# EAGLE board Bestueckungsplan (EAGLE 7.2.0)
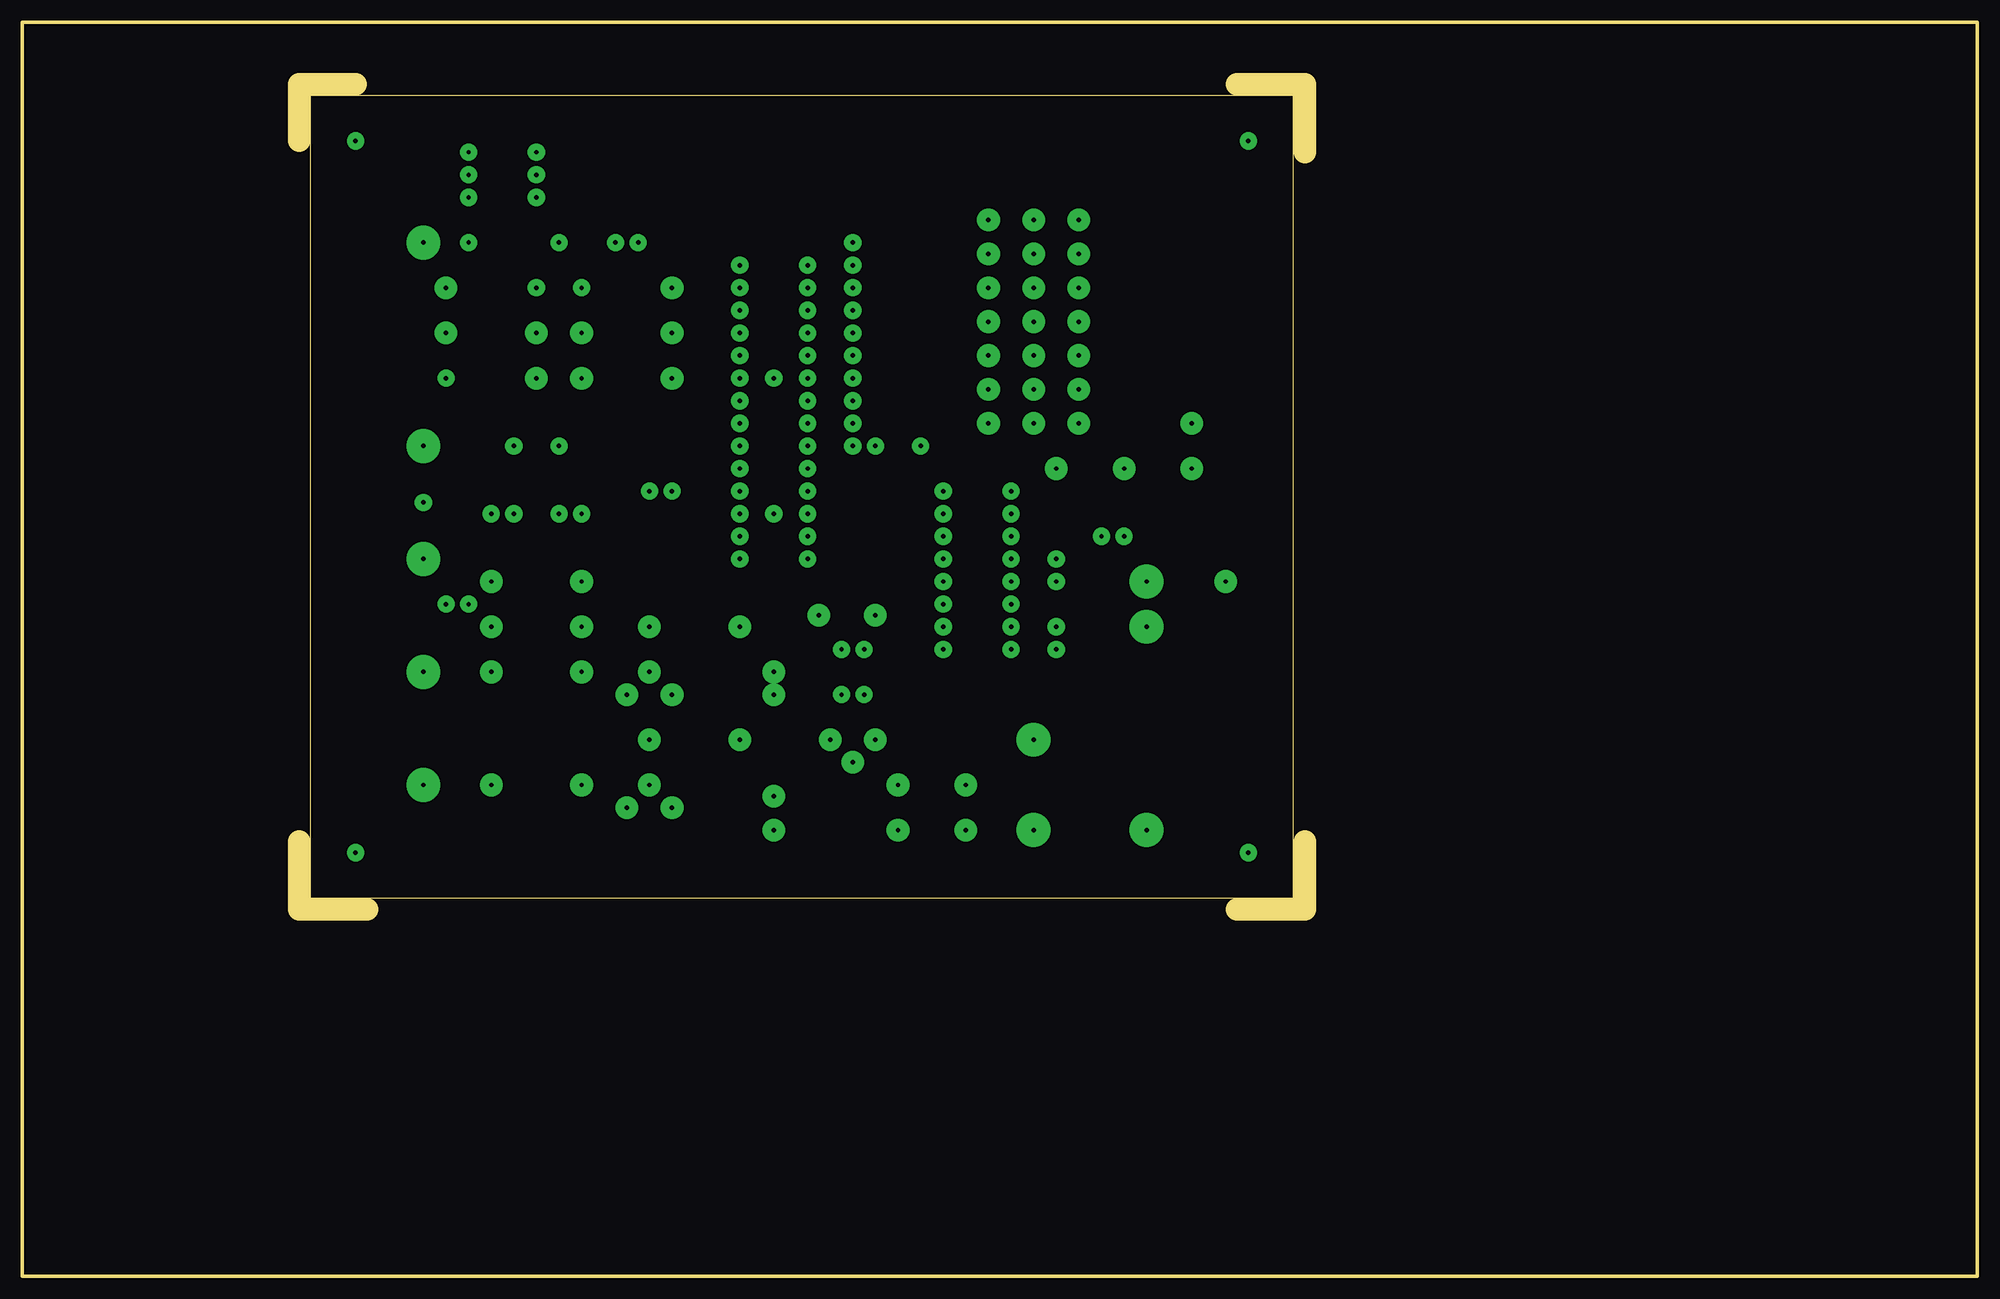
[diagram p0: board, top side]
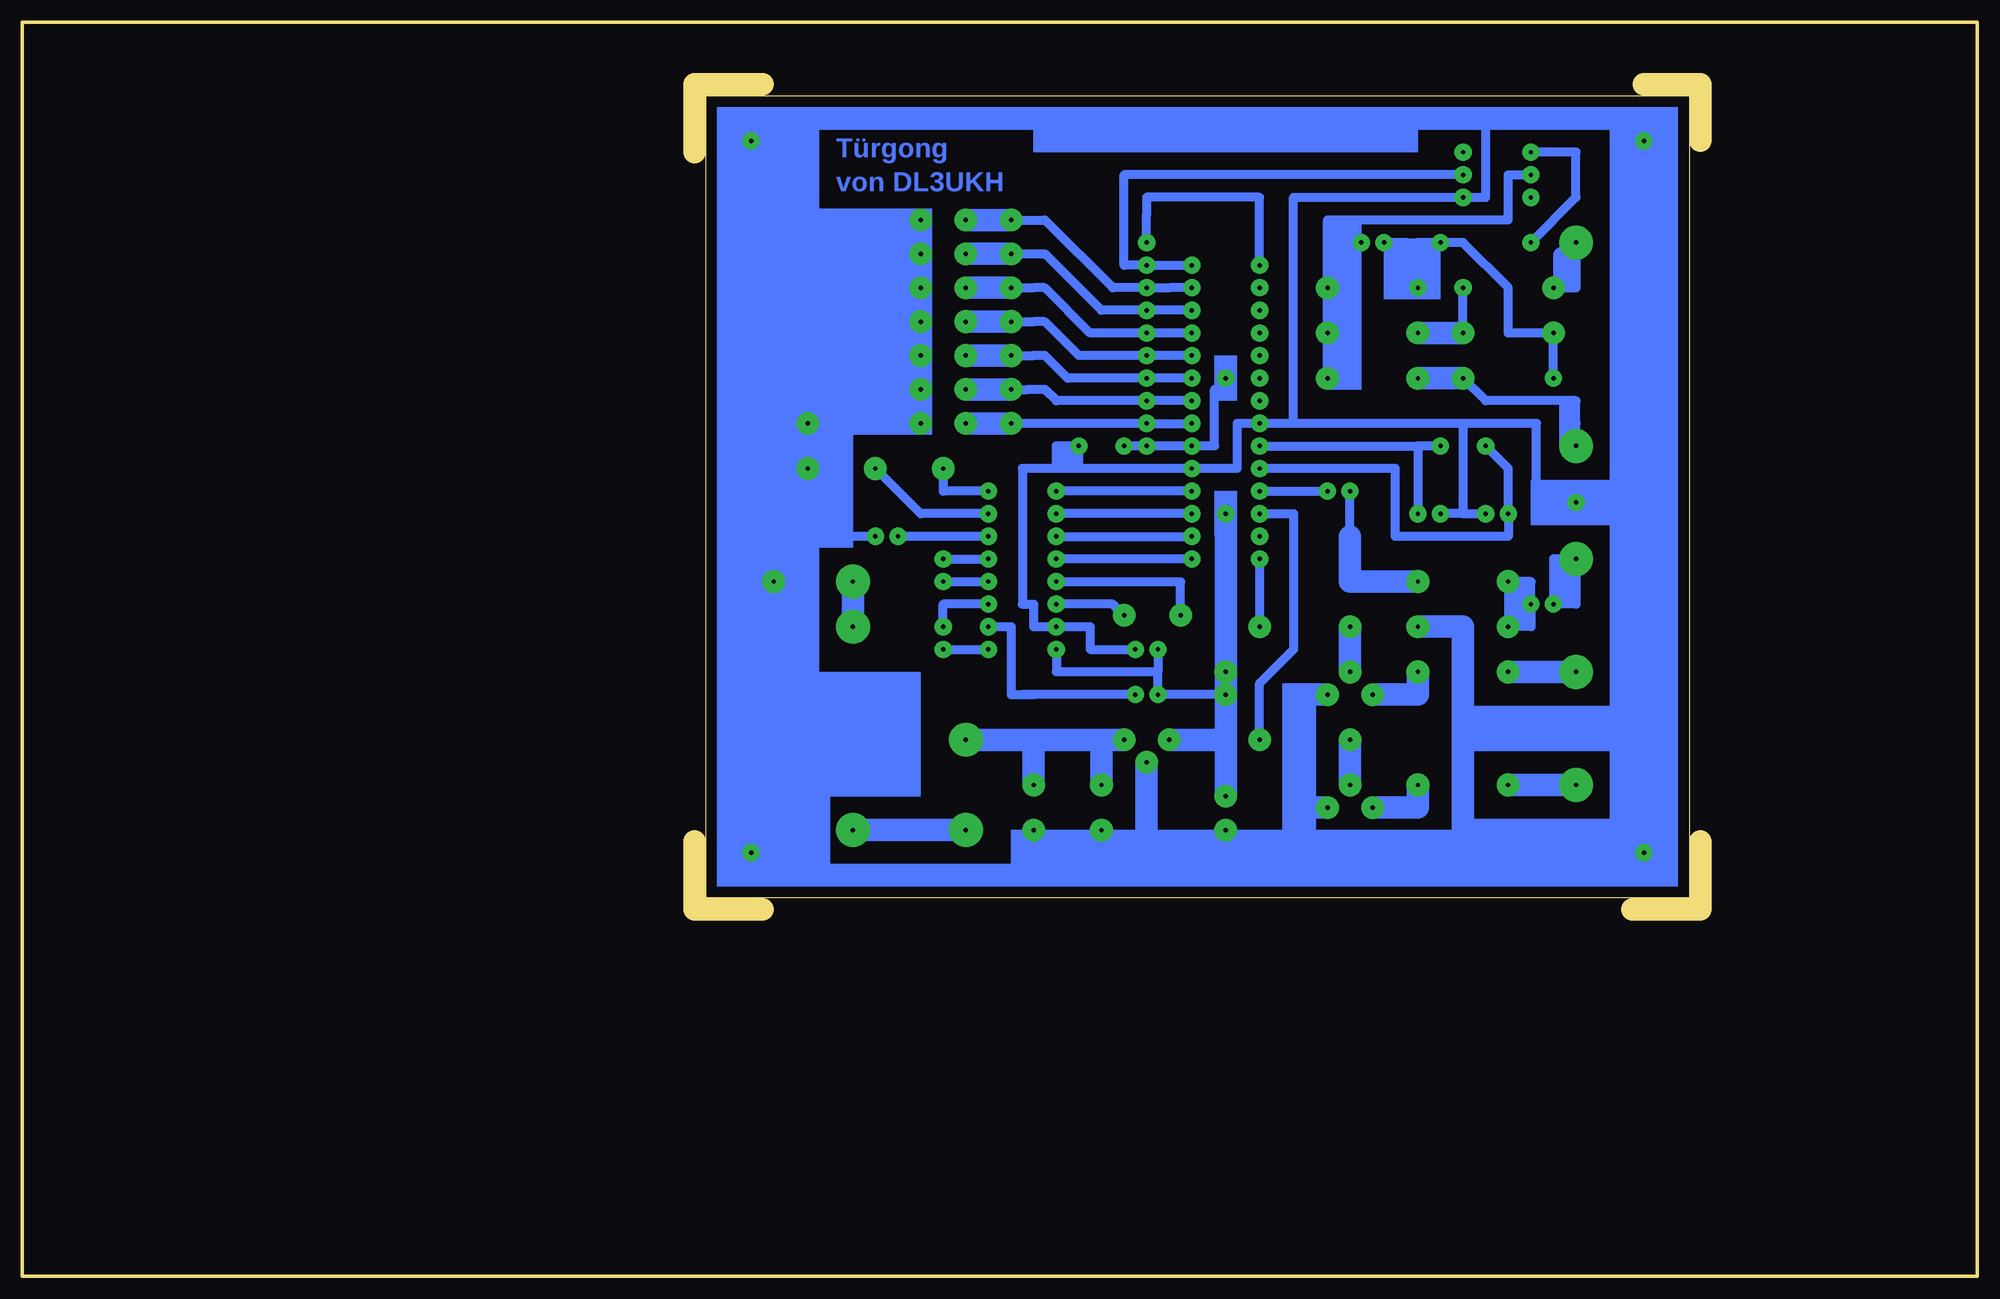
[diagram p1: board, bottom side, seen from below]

Size 219.71 x 140.97 mm. Coordinates in mm from the lower left corner, seen from the top.
Outline: 37.46,133.99 31.11,133.99 31.11,127.64
Outline: 136.53,133.99 144.15,133.99 144.15,126.36
Outline: 31.11,48.9 31.11,41.27 38.73,41.27
Outline: 136.53,41.27 144.15,41.27 144.15,48.9
Outline: 0,140.97 219.71,140.97 219.71,0 0,0 0,140.97
Outline: 32.38,42.55 142.88,42.55 142.88,132.72 32.38,132.72 32.38,42.55
Copper layers (1*16): Top 0.035mm / dielectric 1.5mm / Bottom 0.035mm
Design rules "default": minimum track width 10mil, minimum drill 24mil, track to track 8mil, track to pad 8mil, pad to pad 8mil, via to via 8mil, smd to smd 8mil, copper to edge 40mil, drill to drill 8mil, minimum pad ring 10mil, minimum via ring 8mil, stop-mask expansion 4mil, vias tented up to drill 0mil, thermal gap 10mil

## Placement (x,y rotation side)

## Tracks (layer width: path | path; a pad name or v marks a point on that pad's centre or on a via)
S$1  (via drill 0.5 pad 1.93, 0.5 pad 2.54)
  Bottom 1.016: v80.64,80.65 v80.64,73.03
S$2  (via drill 0.5 pad 1.93)
  other vias: 80.64,83.19
S$3  (via drill 0.5 pad 1.93, 0.5 pad 2.54)
  Bottom 1.016: v80.64,85.72 76.84,85.72 76.84,70.48 80.64,66.67 v80.64,60.33
S$4  (via drill 0.5 pad 2.54, 0.5 pad 3.81)
  Bottom 1.016: v45.08,116.2 45.08,111.12 v47.62,111.12
  Bottom 1.27: v45.08,116.2 46.99,114.94
S$5  (via drill 0.5 pad 1.93)
  Bottom 1.016: v80.64,88.27 v73.03,88.27
S$6  (via drill 0.5 pad 1.93, 0.5 pad 2.54)
  Bottom 1.016: v88.27,100.97 v93.34,100.97 102.23,100.97 104.78,103.5 106.04,103.5 109.22,103.5
  Bottom 2.54: v108.59,103.5 109.22,103.5 v113.66,103.5
S$7  (via drill 0.5 pad 1.93)
  Bottom 1.016: v111.12,73.03 108.59,73.03 108.59,65.41 106.04,65.41 | 106.04,65.41 107.31,65.41 | v94.61,65.41 106.04,65.41
S$8  (via drill 0.5 pad 1.93)
  other vias: 80.64,98.43
S$9  (via drill 0.5 pad 1.93)
  other vias: 80.64,100.97
S$10  (via drill 0.5 pad 1.93)
  other vias: 80.64,103.5
S$11  (via drill 0.5 pad 1.93)
  other vias: 80.64,106.05
S$12  (via drill 0.5 pad 1.93)
  other vias: 80.64,108.59
S$13  (via drill 0.5 pad 1.93)
  other vias: 80.64,111.12
S$14  (via drill 0.5 pad 1.93)
  Bottom 1.016: v80.64,113.67 80.64,121.28 93.34,121.28 93.34,119.38 v93.34,116.2
S$15  (via drill 0.5 pad 1.93)
  Bottom 1.016: v88.27,113.67 v93.34,113.67 95.88,113.67 95.88,123.83 v57.78,123.83
S$16  (via drill 0.5 pad 1.93)
  Bottom 1.016: v88.27,111.12 90.81,111.12 v93.34,111.12
S$17  (via drill 0.5 pad 2.54)
  Bottom 1.016: 93.98,106.05 99.69,106.05 104.78,111.12 106.04,111.12 v108.59,111.12
  Bottom 2.54: v108.59,111.12 v113.66,111.12
S$18  (via drill 0.5 pad 1.93)
  Bottom 1.016: v88.27,106.05 v93.34,106.05
S$19  (via drill 0.5 pad 2.54)
  Bottom 2.54: v70.48,67.94 v70.48,73.03
S$20  (via drill 0.5 pad 1.93, 0.5 pad 2.54)
  Bottom 1.016: 70.48,83.19 v70.48,88.27
  Bottom 2.54: v62.86,78.11 70.48,78.11 70.48,83.19
S$21  (via drill 0.5 pad 2.54)
  Bottom 2.54: v62.86,55.25 62.86,52.7 v67.94,52.7
S$22  (via drill 0.5 pad 1.93, 0.5 pad 2.54)
  Bottom 1.016: v88.27,95.89 v93.34,95.89 v108.59,95.89
  Bottom 2.54: v113.66,95.89 v108.59,95.89
S$23  (via drill 0.5 pad 1.93)
  Bottom 1.016: v95.88,93.34 v93.34,93.34 v88.27,93.34 85.72,93.34 85.72,99.69 84.45,99.69 v84.45,100.97
S$24  (via drill 0.5 pad 1.93, 0.5 pad 2.54)
  Bottom 1.016: v88.27,103.5 v93.34,103.5 100.97,103.5 104.78,107.31 106.04,107.31 v108.59,107.31
  Bottom 2.54: v108.59,107.31 v113.66,107.31
S$25  (via drill 0.5 pad 1.93)
  Bottom 1.016: v88.27,88.27 v103.5,88.27
S$26  (via drill 0.5 pad 1.93)
  Bottom 1.016: v88.27,85.72 v103.5,85.72
S$27  (via drill 0.5 pad 1.93)
  Bottom 1.016: v103.5,83.19 v88.27,83.19
S$28  (via drill 0.5 pad 1.93)
  Bottom 1.016: v88.27,80.65 v103.5,80.65
S$29  (via drill 0.5 pad 1.93, 0.5 pad 2.54)
  Bottom 1.016: v88.27,98.43 v93.34,98.43 103.5,98.43 104.78,99.69 106.68,99.69 v108.59,99.69
  Bottom 2.54: v108.59,99.69 v113.66,99.69
S$30  (via drill 0.5 pad 2.54)
  Bottom 2.54: v70.48,55.25 v70.48,60.33
S$31  (via drill 0.5 pad 2.54, 0.5 pad 3.81)
  Bottom 2.54: v52.7,67.94 v45.08,67.94
S$32  (via drill 0.5 pad 1.93)
  Bottom 1.016: v60.33,93.34 62.86,93.34 | v80.64,93.34 62.86,93.34 | 62.86,93.34 v62.86,85.72
S$33  (via drill 0.5 pad 3.81)
  Bottom 1.016: v126.37,50.16 v113.66,50.16
  Bottom 2.54: v113.66,50.16 v126.37,50.16
S$34  (via drill 0.5 pad 1.93, 0.5 pad 2.54)
  Bottom 1.016: v50.16,75.56 50.16,78.11 v52.7,78.11 v52.7,73.03 50.16,73.03 v50.16,75.56
S$35  (via drill 0.5 pad 2.54)
  Bottom 2.54: v118.75,95.89 v118.75,111.12
S$36  (via drill 0.5 pad 1.93)
  Bottom 1.016: 49.53,87.63 49.53,95.89 57.78,95.89 | v94.61,70.48 99.69,70.48 99.69,73.03 v103.5,73.03 106.04,73.03 106.04,75.56 107.31,75.56 107.31,90.81 103.5,90.81 | 100.97,90.81 v88.27,90.81 83.19,90.81 83.19,95.89 v80.64,95.89 76.84,95.89 | 100.97,90.81 103.5,90.81 | 57.78,85.72 v60.33,85.72 | 57.78,95.89 57.78,85.72 | 57.78,85.72 v55.24,85.72 | 76.84,95.89 76.84,121.28 v57.78,121.28 55.24,121.28 55.24,130.18 | 103.5,90.81 103.5,93.34 v100.97,93.34 100.97,90.81 | 57.78,95.89 76.84,95.89
S$37  (via drill 0.5 pad 1.93)
  other vias: 137.79,47.62
S$38  (via drill 0.5 pad 1.93, 0.5 pad 3.81)
  Bottom 1.016: v45.08,80.65 47.62,80.65 v47.62,75.56 45.08,75.56 v45.08,80.65
S$39  (via drill 0.5 pad 1.93, 0.5 pad 2.54)
  Bottom 1.016: v103.5,78.11 89.53,78.11 v89.53,74.3
S$40  (via drill 0.5 pad 1.93)
  other vias: 137.79,127.64
S$41  (via drill 0.5 pad 2.54)
  other vias: 118.75,99.69
S$42  (via drill 0.5 pad 1.93)
  Bottom 1.016: v116.2,70.48 v111.12,70.48
S$43  (via drill 0.5 pad 1.93, 0.5 pad 2.54)
  Bottom 1.016: v118.75,103.5 128.91,106.05 128.91,83.19 v123.82,83.19
S$44  (via drill 0.5 pad 1.93)
  Bottom 1.016: v111.12,75.56 116.2,75.56 v116.2,73.03
S$45  (via drill 0.5 pad 1.93)
  Bottom 1.016: v116.2,78.11 v111.12,78.11
S$46  (via drill 0.5 pad 1.93)
  Bottom 1.016: v116.2,80.65 v111.12,80.65
S$47  (via drill 0.5 pad 1.93)
  Bottom 1.016: v111.12,83.19 v121.28,83.19
S$48  (via drill 0.5 pad 1.93, 0.5 pad 2.54)
  Bottom 1.016: v111.12,85.72 118.75,85.72 v123.82,90.81
S$49  (via drill 0.5 pad 1.93, 0.5 pad 2.54)
  Bottom 1.016: v116.2,90.81 116.2,88.27 v111.12,88.27
S$50  (via drill 0.5 pad 2.54)
  other vias: 118.75,107.31
S$51  (via drill 0.5 pad 2.54)
  Bottom 1.016: 93.98,111.12 97.16,111.12 104.78,118.75 v108.59,118.75
  Bottom 2.54: v108.59,118.75 110.49,118.75 v113.66,118.75
S$52  (via drill 0.5 pad 3.81)
  Bottom 2.54: v126.37,73.03 v126.37,78.11
S$53  (via drill 0.5 pad 1.93)
  Bottom 1.016: v55.24,93.34 52.7,90.81 v52.7,85.72 52.7,83.19 65.41,83.19 65.41,90.81 v80.64,90.81
S$54  (via drill 0.5 pad 1.93)
  other vias: 57.78,126.36
S$55  (via drill 0.5 pad 1.93, 0.5 pad 2.54)
  Bottom 1.016: v50.16,123.83 52.7,123.83 52.7,118.75 73.03,118.75 73.03,114.94 | v69.22,116.2 73.03,116.2 73.03,114.94 | 73.03,114.94 v73.03,111.12 v73.03,106.05 v73.03,100.97
S$56  (via drill 0.5 pad 2.54, 0.5 pad 3.81)
  Bottom 2.54: v52.7,55.25 v45.08,55.25
S$57  (via drill 0.5 pad 2.54)
  other vias: 131.44,90.81
S$58  (via drill 0.5 pad 2.54)
  Bottom 2.54: v62.86,67.94 62.86,65.41 v67.94,65.41
S$59  (via drill 0.5 pad 1.93)
  other vias: 37.46,47.62
S$60  (via drill 0.5 pad 1.93, 0.5 pad 2.54)
  Bottom 1.016: v84.45,67.94 v84.45,85.72 | v84.45,65.41 v92.07,65.41 92.07,67.94 | v92.07,70.48 92.07,67.94 | 92.07,67.94 103.5,67.94 v103.5,70.48
  Bottom 2.54: v84.45,85.72 v84.45,67.94 v84.45,65.41 84.45,60.33 | 84.45,60.33 v84.45,53.98 | 84.45,60.33 v90.81,60.33
S$61  (via drill 0.5 pad 1.93)
  other vias: 50.16,121.28
S$62  (via drill 0.5 pad 1.93, 0.5 pad 2.54)
  Bottom 1.016: v95.88,74.3 97.16,75.56 v103.5,75.56
S$63  (via drill 0.5 pad 1.93)
  other vias: 37.46,127.64
S$64  (via drill 0.5 pad 2.54, 0.5 pad 3.81)
  Bottom 1.016: 98.43,60.33 106.04,60.33
  Bottom 2.54: v98.43,55.25 98.43,60.33 v95.88,60.33 106.04,60.33 | v113.66,60.33 106.04,60.33 | 106.04,60.33 v106.04,55.25
S$65  (via drill 0.5 pad 2.54)
  Bottom 1.016: 57.78,47.62 75.56,47.62 84.45,47.62 93.34,47.62 98.43,47.62 | v106.04,50.16 106.04,47.62 98.43,47.62 | v98.43,50.16 98.43,47.62
  Bottom 2.54: v93.34,57.79 93.34,47.62 | v98.43,50.16 98.43,46.36 | v106.04,50.16 106.04,46.36 | v73.03,65.41 75.56,65.41 75.56,52.7 | 75.56,47.62 75.56,52.7 | 75.56,52.7 v73.03,52.7 | v62.86,73.03 57.78,73.03 57.78,47.62 | v84.45,50.16 84.45,47.62
S$66  (via drill 0.5 pad 2.54)
  other vias: 135.25,78.11
S$67  (via drill 0.5 pad 2.54)
  other vias: 131.44,95.89
S$68  (via drill 0.5 pad 1.93)
  other vias: 45.08,87
S$73  (via drill 0.5 pad 1.93)
  Bottom 1.016: v50.16,126.36 45.08,126.36 45.08,121.28 v50.16,116.2
S$75  (via drill 0.5 pad 1.93, 0.5 pad 2.54)
  Bottom 1.016: v57.78,106.05 v57.78,111.12
  Bottom 2.54: v57.78,106.05 60.33,106.05 v62.86,106.05
S$76  (via drill 0.5 pad 2.54, 0.5 pad 3.81)
  Bottom 1.016: 45.08,95.89 v45.08,93.34 45.08,98.43 55.24,98.43 v57.78,100.97 v62.86,100.97
  Bottom 2.54: v57.78,100.97 v62.86,100.97
S$78  (via drill 0.5 pad 1.93, 0.5 pad 2.54)
  Bottom 1.016: v47.62,100.97 v47.62,106.05 52.7,106.05 52.7,111.12 57.78,116.2 v60.33,116.2 62.86,116.2 | v66.67,116.2 64.13,116.2 62.86,116.2 | v62.86,111.12 62.86,116.2
S$81  (via drill 0.5 pad 1.93, 0.5 pad 2.54)
  Bottom 1.016: v88.27,108.59 v93.34,108.59 98.43,108.59 104.78,114.94 v108.59,114.94
  Bottom 2.54: v108.59,114.94 110.49,114.94 v113.66,114.94
S$83  (via drill 0.5 pad 2.54)
  other vias: 118.75,114.94
S$84  (via drill 0.5 pad 2.54)
  other vias: 118.75,118.75
(copper drawn outside any net)
  shapes: Bottom area x34

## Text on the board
Bottom: Türgong | von DL3UKH
tOrigins: BOHRUNGEN | Leiterplatte: | alles 0.8mm | 1,5mm dick | Diode 1N4002 1,0mm | Cevausit | Sicherungshalter 1,5mm | 1 | 6 | Anschluß-Drähte 1,0mm | 4Stck. Befestigungsbohr... 3,2mm | 3 | 4 | CNY17 | Einzel / 24h Melodie Schal. | Klingeldruckspannung | 1K | 1 | 28 | 22µ/63V | Melodie-Wiederholungs Schal. | 1K | 10K | Melodieauswahl Schal. | Kat | Melodieauswahl Schal. | Kat | PIC16F876 | 4x 1N4148 | Melodieauswahl Schal. | 78L05 | 7x 47n | Kat | Brücke | 9x 10K | 7x Schalter | Melodieauswahl Schal. | Kat | 4Mhz | Melodieauswahl Schal. | Klingeldruckspannung | Pin3 | Pin2 | 47n | 10µ/35V | 8 | SUB-D Masse | Pin5 | 9 | NF-Masse | 1µ/Tant. | 15p | 15p | Speisespannung | +14 Volt | NF-Ausgang | 14 | 15 | Ausg. | Eing. | 100K | Masse | Pin7 | Pin8 | Masse | 1,5K | 15K | 10µ/35V | MAX232CPE | +5V | 16 | 1 | Steht für den | BC547c | Kontroll-LED | 220 | E | 2x 1µ/Tant. | 2x 1µ/Tant. | Pluspol eines | +5V | BC547c | µA78L05 | Kat | Elkos oder | Eing. | 7,5K | Tantal-Kond. | + ist immer | 5 Volt Relais | Brücke | E | langer Draht | 47n | 1N4002 | Sicherungshalter | Die zwei Brücken | BC547c | wenn bei Tantal | nicht vergessen! | beide Drähte | 220µ/16V | 220µ/35V | mit 250mA Sicherung | C | E | gleich sind ist | B | grüne 5mm LED | es egal | (ohne Fassung dargestellt) | Widerstandsnetzwerk 9x10K | Sub-D-Stecker | 1N4002 + 1N4148 | 15K | von hinten auf die Löt- | IC's | 1 | anschlüsse gesehen. | Links oben ist | Pin5 | Pin1 | immer PIN 1 | Der Punkt auf dem Bauelement muß | langer | mit dem Punkt auf dem Bestückungs- | Katode | Anode | Anschluß- | plan hier übereinstimmen, so daß das | mit Kat | draht | Bauelement richtig herum eingelötet | gekennzeichnet | an +5V | wird. | hier im Plan | Pin9 | Pin6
